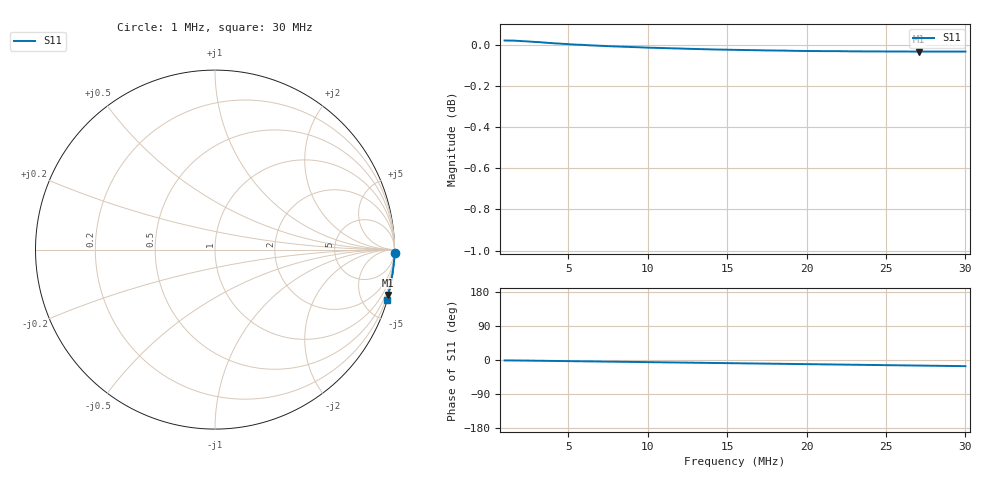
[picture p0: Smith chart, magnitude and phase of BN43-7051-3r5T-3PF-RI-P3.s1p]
! ListType=Log
!!BN43-7051 3.5T 3PF Port 3
# MHz S RI R 50
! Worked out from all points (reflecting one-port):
!   101 points, 1 MHz to 30 MHz, reference 50 ohm
!   lowest |S11| = 0.0 dB at 27.09 MHz (marker M1), VSWR 534.93, Z = 5.71 - j387 ohm
!   phase of S11 starts at -1 deg and turns -15 deg over the sweep
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1  1.002 -0.0189
1.107423  1.002 -0.0192
1.185376  1.002 -0.0194
1.358129  1.002 -0.0202
1.66559  1.002 -0.0222
2.042657  1.002 -0.0251
2.421316  1.002 -0.0283
2.87017  1.001 -0.0322
3.178493  1.001 -0.035
3.519937  1.001 -0.0381
4.780527  0.9993 -0.0496
5.666721  0.9984 -0.0578
5.862773  0.9983 -0.0596
8.52288  0.9954 -0.0842
9.438436  0.9944 -0.0925
11.97563  0.9912 -0.1159
13.72092  0.9888 -0.1319
15.72057  0.9858 -0.1501
16.82715  0.9841 -0.1602
18.01163  0.9821 -0.171
19.27949  0.9798 -0.1825
22.08922  0.9746 -0.2079
22.85344  0.973 -0.2148
23.6441  0.9713 -0.2219
25.30843  0.9677 -0.2369
27.08991  0.9636 -0.2529
28.9968  0.959 -0.2699
30  0.9564 -0.2789
